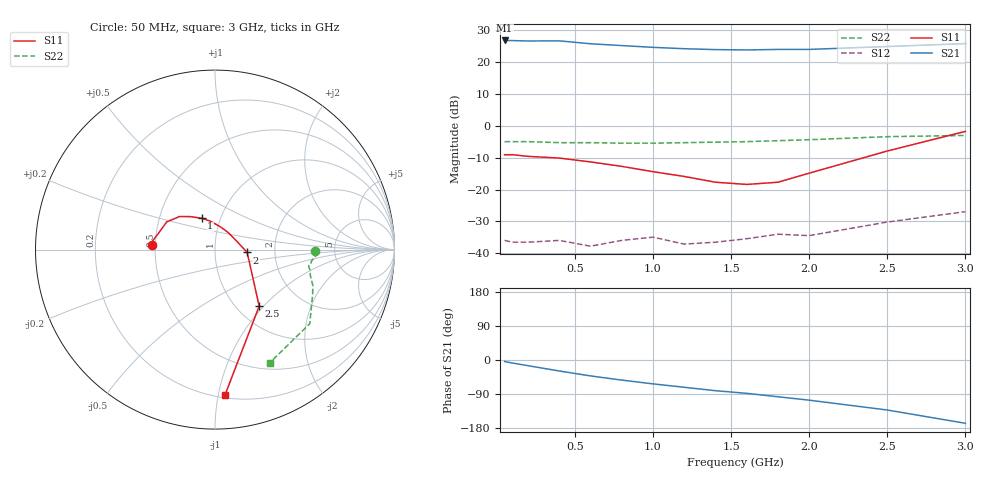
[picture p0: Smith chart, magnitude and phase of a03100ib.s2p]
!  INA-03100  S PARAMETERS
!  Id = 12 mA  LAST UPDATED 06-23-94
# ghz s ma r 50
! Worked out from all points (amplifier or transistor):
!   14 points, 50 MHz to 3 GHz, reference 50 ohm
!   highest |S21| = 26.6 dB at 50 MHz (marker M1)
!   |S21| within 3 dB of that: start of sweep to end of sweep
!   unconditionally stable (mu >= 1): start of sweep to 2.118 GHz
!   at 200 MHz: K = 1.31, MAG = 28.1 dB, |S12| = -36.5 dB
!   at 1.2 GHz: K = 1.75, MAG = 25.5 dB, |S12| = -37.1 dB
!   at 3 GHz: K = 0.04, MSG = 26.3 dB, |S12| = -26.9 dB
!   S11 on the Smith chart (normalised r, x): 50 MHz: 0.48, +0.03; 1 GHz: 0.81, +0.30; 2 GHz: 1.44, -0.05; 2.5 GHz: 1.26, -0.94; 3 GHz: 0.22, -1.05
0.05  0.35 176.0  21.4 -4.0  0.016 8.0  0.56 -1.0
0.1  0.35 172.0  21.3 -8.0  0.015 -4.0  0.56 -3.0
0.2  0.33 165.0  21 -15.0  0.015 -5.0  0.56 -4.0
0.4  0.31 150.0  21.1 -29.0  0.016 -13.0  0.54 -7.0
0.6  0.27 137.0  19 -42.0  0.013 -14.0  0.54 -8.0
0.8  0.23 127.0  17.8 -53.0  0.016 -13.0  0.53 -9.0
1  0.19 113.0  16.7 -63.0  0.018 -16.0  0.53 -10.0
1.2  0.16 99.0  15.9 -72.0  0.014 -21.0  0.54 -12.0
1.4  0.13 76.0  15.4 -81.0  0.015 -12.0  0.55 -15.0
1.6  0.12 51.0  15.2 -88.0  0.017 -11.0  0.56 -17.0
1.8  0.13 21.0  15.5 -97.0  0.02 -5.0  0.58 -20.0
2  0.18 -5.0  15.5 -106.0  0.019 -13.0  0.6 -25.0
2.5  0.4 -52.0  17.2 -132.0  0.031 -9.0  0.67 -38.0
3  0.81 -86.0  19.1 -167.0  0.045 -12.0  0.7 -64.0
